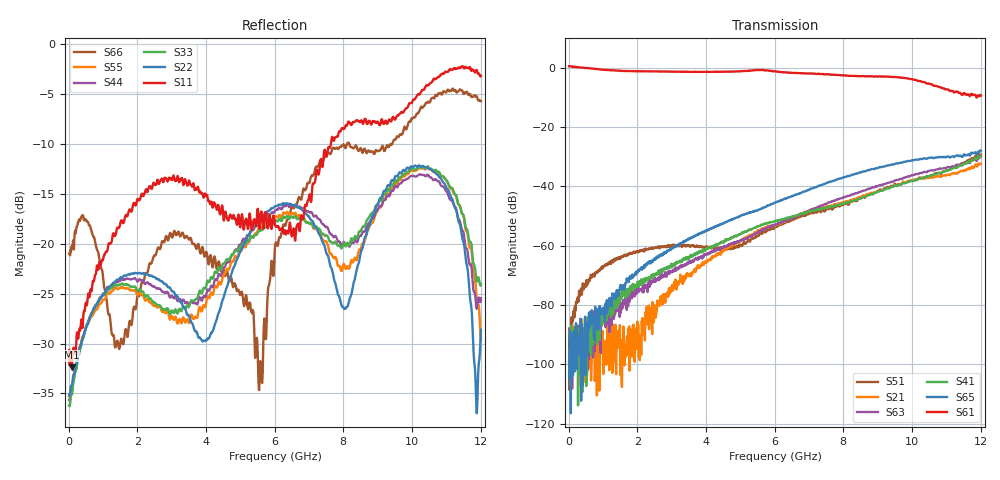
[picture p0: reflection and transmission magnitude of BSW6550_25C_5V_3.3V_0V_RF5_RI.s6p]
! Agilent Technologies	N5230C	MY49001333	A.09.33.09
!	Test time	=	2026-05-06 10:00
!	Product	=	BSW6550
!	Temp	=	25C
!	VDD	=	5
!	Control_High	=	3.3
!	Control_Low	=	0
!	Logic	=	RF5
!	Port1	=	RFC
!	Port2	=	RF1
!	Port3	=	RF2
!	Port4	=	RF3
!	Port5	=	RF4
!	Port6	=	RF5
!	V1	=	3.3 / 0
!	V2	=	3.3 / 0
!	V3	=	3.3 / 0
!S6P File: Measurements: <S11,S12,S13,S14,S15,S16>,
!<S21,S22,S23,S24,S25,S26>,
!<S31,S32,S33,S34,S35,S36>,
!<S41,S42,S43,S44,S45,S46>,
!<S51,S52,S53,S54,S55,S56>,
!<S61,S62,S63,S64,S65,S66>;
# HZ S RI R 50
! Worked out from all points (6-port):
!   1201 points, 10 MHz to 12.01 GHz, reference 50 ohm
!   strongest paths, dB at 10 MHz, 3.01 GHz, 6.01 GHz, 9.01 GHz, 12.01 GHz:
!     S61: 0.5, -1.3, -1.2, -3.0, -9.4
!     S65: -97.6, -60.9, -45.5, -33.8, -28.0
!     S41: -99.1, -66.6, -51.6, -41.8, -29.8
!     S63: -87.9, -69.0, -52.9, -39.9, -30.0
!     S21: -104.1, -74.3, -53.2, -41.7, -32.4
!     S51: -99.2, -60.0, -53.4, -41.6, -29.3
!   lowest |S11| = -32.4 dB at 90 MHz (marker M1), VSWR 1.05, Z = 52.4 - j0.519 ohm
!   |S11| at or under -10 dB: start of sweep to 7.638 GHz
